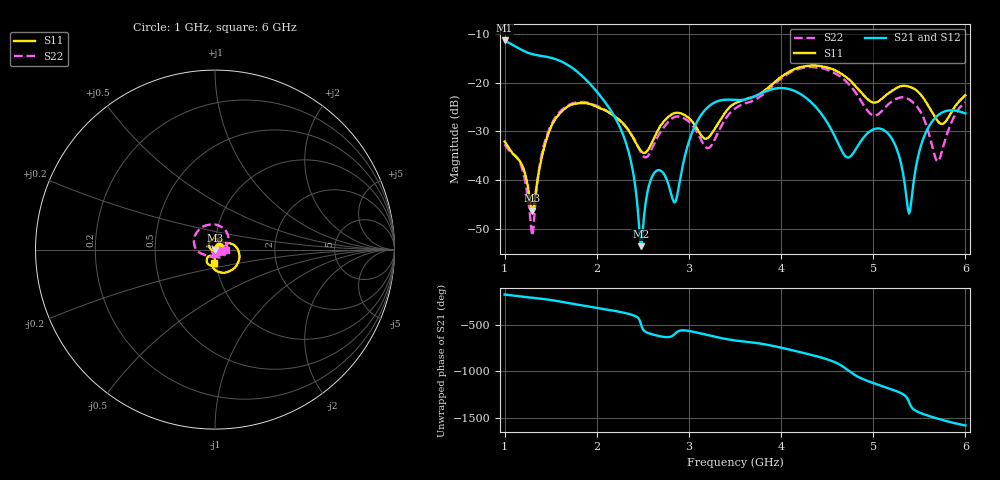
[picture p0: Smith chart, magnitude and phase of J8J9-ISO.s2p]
!Agilent Technologies,E8364B,MY43040528,A.07.50.67
!Agilent E8364B: A.07.50.67
!Date: Sunday, March 01, 2026 23:22:46
!Correction: S11(Full 2 Port(1,2))
!S21(Full 2 Port(1,2))
!S12(Full 2 Port(1,2))
!S22(Full 2 Port(1,2))
!S2P File: Measurements: S11, S21, S12, S22:
# Hz S  dB  R 50
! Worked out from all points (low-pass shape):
!   451 points, 1 GHz to 6 GHz, reference 50 ohm
!   highest |S21| = -11.39 dB at 1 GHz (marker M1); lowest = -53.5 dB at 2.478 GHz (marker M2)
!   |S21| within 3 dB of the highest: start of sweep to 1.348 GHz
!   lowest |S11| = -46.3 dB at 1.3 GHz (marker M3), VSWR 1.01, Z = 50.2 - j0.449 ohm
!   |S11| at or under -10 dB: start of sweep to end of sweep
!   |S22| runs from -51.4 to -16.8 dB; largest |S21 - S12| = 0.0011
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1e9  -32.09 32.2  -11.39 -166.8  -11.42 -166.8  -32.64 -13.4
1.177778e9  -36.50 20.0  -13.25 172.1  -13.28 172.1  -36.96 -25.1
1.3e9  -46.27 -67.0  -14.19 159.9  -14.22 160.0  -51.38 -132.4
1.477778e9  -30.31 161.4  -14.82 137.5  -14.85 137.5  -29.89 87.8
1.844444e9  -24.21 79.9  -18.72 74.8  -18.74 74.8  -23.98 -9.0
2.288889e9  -28.45 26.2  -30.87 -2.6  -30.89 -2.6  -28.53 -87.3
2.388889e9  -31.15 21.9  -37.84 -28.7  -37.88 -28.8  -30.98 -99.6
2.477778e9  -33.97 33.0  -53.52 -121.3  -53.62 -121.2  -34.28 -95.1
2.566667e9  -33.50 60.9  -41.11 132.6  -41.15 132.7  -34.76 -72.4
2.666667e9  -29.67 68.1  -37.95 105.0  -37.98 105.1  -30.90 -64.7
2.844444e9  -26.27 45.5  -44.57 124.0  -44.60 124.0  -27.05 -97.7
3.111111e9  -30.20 21.1  -27.28 135.1  -27.32 135.1  -31.00 -143.4
3.222222e9  -31.09 43.5  -24.78 109.1  -24.81 109.1  -33.33 -124.9
3.5e9  -24.27 43.4  -23.57 55.8  -23.61 55.8  -25.35 -130.6
4.344444e9  -16.51 -39.5  -24.38 -105.1  -24.42 -105.1  -16.85 111.3
4.711111e9  -18.96 -90.1  -35.28 103.7  -35.32 103.7  -19.89 42.5
4.988889e9  -24.04 -93.7  -29.70 -41.9  -29.74 -41.9  -26.64 28.9
5.166667e9  -22.19 -85.4  -30.58 -103.4  -30.61 -103.4  -24.40 34.1
5.388889e9  -20.86 -111.6  -46.84 106.6  -46.89 106.7  -23.46 -7.0
5.522222e9  -22.63 -128.8  -32.65 -14.3  -32.69 -14.3  -26.29 -35.1
5.7e9  -27.91 -122.6  -26.75 -72.2  -26.79 -72.2  -36.16 -11.3
6e9  -22.60 -95.3  -26.35 -145.9  -26.39 -145.9  -24.06 -3.4
